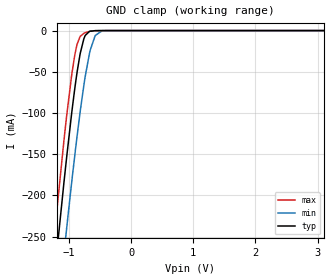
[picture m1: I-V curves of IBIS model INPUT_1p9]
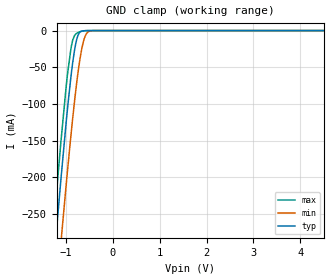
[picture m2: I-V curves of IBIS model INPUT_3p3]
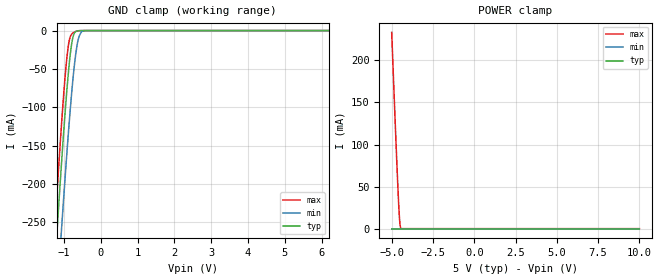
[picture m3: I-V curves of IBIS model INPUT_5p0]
|Texas Instruments Incorporated
|DACx3608, Octal, 10-Bit or 8-Bit, I2C Interface, Buffered Voltage Output
|DACs in Tiny 3 * 3 QFN Package
[IBIS Ver]   4.1
[File name]   dac43608.ibs
[Date]   11/02/2018
[File Rev]   1.0
[Source]
| Texas Instruments Incorporated.
| Analog-eLab Design Center, HPA
| 12500 TI Blvd
| Dallas, TX -75243
[Notes]   Revision History:
| Rev 1.0: 11/02/2018
| - Initial version of the model
| - Model generated from simulations in SPECTRE
|   Model names with a trailing _1p9 contain the model for 1.9V operation.
|   Model names with a trailing _3p3 contain the model for 3.3V operation.
|   Model names with a trailing _5p0 contain the model for 5.0V operation.
| - C_comp although listed in numerical order of value are
|   obtained from varying PVT conditions. For PVT conditions for
|   each specific value refer the buffer description under
|   respective [Model]. IBIS model user is responsible for using
|   appropriate C_comp to simulate for Signal Integrity.
| - Warnings regarding combined Non-monotonicity of various models
|   have been reviewed and considered minor and can be ignored.
[Disclaimer]
| This model is designed as an aid for customers of Texas Instruments.
| TI and its licensors and suppliers make no warranties, either expressed
| or implied, with respect to this  model, including the warranties of
| merchantability or fitness for a particular purpose. The model is
| provided solely on an "as is" basis. The entire risk as to its quality
| and performance is with the customer.
| This model is subject to change without notice. Texas Instruments
| Incorporated is not responsible for updating this model.
[Copyright]
(C) Copyright 2018 Texas Instruments Incorporated.All rights reserved.
|  Component DAC43608RTE 16-pin WQFN - RTE package
|  Part # DAC43608RTE
[Component]   DAC43608RTE
[Manufacturer]  TI
[Package]   |16-pin WQFN - RTE package
|   typ   min   max
R_pkg   0.05   0.04   0.06
L_pkg   1.0nH   0.8nH   1.2nH
C_pkg   0.2pF   0.16pF   0.24pF
[Pin]   signal_name   model_name   R_pin   L_pin   C_pin
1   VOUTA   NC   NA   NA   NA
2   VOUTB   NC   NA   NA   NA
3   VOUTC   NC   NA   NA   NA
4   VOUTD   NC   NA   NA   NA
5   SDA   IO_OPENDRAIN   NA   NA   NA
6   SCL   INPUT   NA   NA   NA
7   A0   INPUT   NA   NA   NA
8   LDACb   INPUT   NA   NA   NA
9   VOUTE   NC   NA   NA   NA
10   VOUTF   NC   NA   NA   NA
11   VOUTG   NC   NA   NA   NA
12   VOUTH   NC   NA   NA   NA
13   VDD   POWER   NA   NA   NA
14   AGND   GND   NA   NA   NA
15   VREFIN   NC   NA   NA   NA
16   CLRb   INPUT   NA   NA   NA
|   Model Selectors
[Model Selector] IO_OPENDRAIN
OPENDRAIN_1p9  1.9V   digital I/O_open_drain
OPENDRAIN_3p3  3.3V   digital I/O_open_drain
OPENDRAIN_5p0  5.0V   digital I/O_open_drain
[Model Selector] INPUT
INPUT_1p9   1.9V   digital Input
INPUT_3p3   3.3V   digital Input
INPUT_5p0   5.0V   digital Input
| Models and submodels in the file (6): INPUT_1p9 (Input), INPUT_3p3 (Input), INPUT_5p0 (Input), OPENDRAIN_1p9 (I/O_open_drain), OPENDRAIN_3p3 (I/O_open_drain), OPENDRAIN_5p0 (I/O_open_drain)
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|   INPUT_1p9 Model
[Model]   INPUT_1p9
Model_type   Input
Vinl = 0.5
Vinh = 1.6
|   typ   min   max
C_comp   1.643E-12   1.620E-12   1.674E-12
|  Where Nom  PVT is Nominal Process, 1.9V,   25C
|   Fast PVT is Strong Process,  2.0V,  -40C
|   Slow PVT is Weak Process,   1.8V,  125C
[Voltage Range]   1.9   1.8   2
|Junction Temperature
[Temperature Range]   25   125   -40
[Power Clamp Reference]   1.9   1.8   2
[GND Clamp Reference]   0   0   0
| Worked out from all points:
|   GND clamp passes 1 mA (typ) near -0.67 V on its own axis
[GND Clamp]
|   Voltage   I(typ)   I(min)   I(max)
-1.9V     -827.7mA   -896.1mA   -789.8mA
-1.227V   -292.9mA   -378.3mA   -242.6mA
-1.079V   -183.4mA   -269.9mA   -132.5mA
-1.034V   -151.5mA   -237.6mA   -101.3mA
-953.8mV  -98.83mA   -182.9mA   -52.93mA
-885.4mV  -58.93mA   -138.4mA   -22mA
-822.7mV  -29.4mA    -100.3mA   -7.507mA
-760mV    -9.878mA   -66.25mA   -3.337mA
-657.4mV  -734.5uA   -23.67mA   -758uA
-577.6mV  -103.2uA   -6.026mA   -131.6uA
-469.3mV  -6.097uA   -376.1uA   -5.993uA
3.8V      0A         0A         0A
[POWER Clamp]
|   Voltage   I(typ)   I(min)   I(max)
-1.9V     0A         0A         0A
0V        0A         0A         0A
3.8V      0A         0A         0A
|   INPUT_3p3 Model
[Model]   INPUT_3p3
Model_type   Input
Vinl = 0.5
Vinh = 2.4
|   typ   min   max
C_comp   1.498E-12   1.471E-12   1.519E-12
|  Where Nom  PVT is Nominal Process, 3.3V,   25C
|   Fast PVT is Strong Process,  3.6V,  -40C
|   Slow PVT is Weak Process,   3.0V,  125C
[Voltage Range]   3.3   3   3.6
|Junction Temperature
[Temperature Range]   25   125   -40
[Power Clamp Reference]   3.3   3   3.6
[GND Clamp Reference]   0   0   0
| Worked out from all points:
|   GND clamp passes 1 mA (typ) near -0.67 V on its own axis
[GND Clamp]
|   Voltage   I(typ)   I(min)   I(max)
-3.3V     -1.941A    -1.934A    -1.954A
-1.27V    -325.9mA   -410.5mA   -276.2mA
-1.251V   -310.7mA   -395.7mA   -260.7mA
-1.191V   -265.7mA   -351.5mA   -214.9mA
-1.102V   -199.9mA   -286.4mA   -148.8mA
-983.4mV  -117.8mA   -202.9mA   -69.72mA
-894.3mV  -63.74mA   -144mA     -25.25mA
-795.3mV  -19.44mA   -84.87mA   -5.089mA
-726mV    -4.381mA   -50.01mA   -2.204mA
-607.2mV  -213.1uA   -10.84mA   -267.4uA
-468.6mV  -5.966uA   -368.8uA   -5.846uA
6.6V      0A         0A         0A
[POWER Clamp]
|   Voltage   I(typ)   I(min)   I(max)
-3.3V     0A         0A         0A
0V        0A         0A         0A
6.6V      0A         0A         0A
|   INPUT_5p0 Model
[Model]   INPUT_5p0
Model_type   Input
Vinl = 0.5
Vinh = 2.4
|   typ   min   max
C_comp   1.386E-12   1.367E-12   1.398E-12
|  Where Nom  PVT is Nominal Process, 5.0V,   25C
|   Fast PVT is Strong Process,  5.5V,  -40C
|   Slow PVT is Weak Process,   4.5V,  125C
[Voltage Range]   5   4.5   5.5
|Junction Temperature
[Temperature Range]   25   125   -40
[Power Clamp Reference]   5   4.5   5.5
[GND Clamp Reference]   0   0   0
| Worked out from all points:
|   GND clamp passes 1 mA (typ) near -0.67 V on its own axis
[GND Clamp]
|   Voltage   I(typ)   I(min)   I(max)
-5V       -3.241A    -3.165A    -3.308A
-1.25V    -310.2mA   -395.2mA   -260.2mA
-1.235V   -298.7mA   -383.9mA   -248.5mA
-1.145V   -231.2mA   -317.4mA   -180.1mA
-1.07V    -176.9mA   -263.3mA   -126.1mA
-920mV    -78.33mA   -160.5mA   -36.05mA
-860mV    -45.97mA   -122.6mA   -14.3mA
-800mV    -21mA      -87.47mA   -5.409mA
-680mV    -1.31mA    -31.29mA   -1.125mA
-590mV    -139.9uA   -7.8mA     -178.4uA
-410mV    -1.035uA   -70.95uA   -709.1nA
10V       0A         0A         0A
[POWER Clamp]
|   Voltage   I(typ)   I(min)   I(max)
-5V       1.428nA    3.532nA    233.3mA
-4.85V    0A         0A         157.2mA
-4.745V   0A         0A         105.3mA
-4.655V   0A         0A         62.67mA
-4.595V   0A         0A         36.39mA
-4.55V    0A         0A         19.18mA
-4.52V    0A         0A         10.06mA
-4.505V   0A         0A         6.584mA
-4.475V   0A         0A         2.219mA
-4.43V    0A         0A         282.9uA
10V       0A         0A         0A
